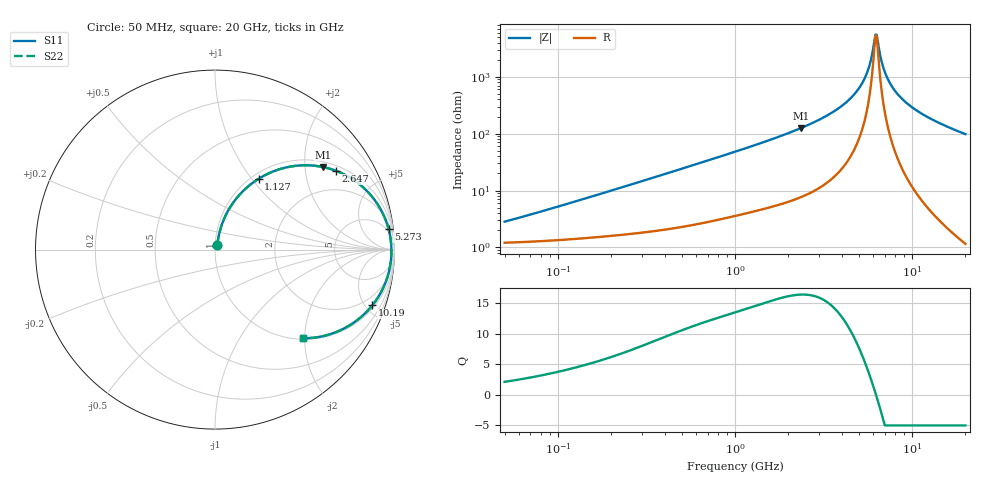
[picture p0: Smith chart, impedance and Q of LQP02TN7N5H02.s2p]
!Murata Part Number: LQP02TN7N5H02
!These Parameters are Measured in Series Mode Connection
!  o--[Z]--o
!Port1  Port2
!  o-------o
!Freq. Start=50[MHz] Stop=20[GHz], 401[Steps]
# Hz S RI R 50
!Freq.(Hz) S11(Real) S11(Imag) S21(Real) S21(Imag) S12(Real) S12(Imag) S22(Real) S22(Imag)
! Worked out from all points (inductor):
!   401 points, 50 MHz to 20 GHz, reference 50 ohm
!   read as one part in series: L = 8.03 nH near 76.05 MHz
!   highest Q = 16.4 at 2.349 GHz (marker M1), where L = 8.44 nH
!   self-resonance near 6.218 GHz
!   S11 on the Smith chart (normalised r, x): 50 MHz: 1.02, +0.05; 1.127 GHz: 1.08, +1.08; 2.647 GHz: 1.18, +2.93; 5.273 GHz: 4, +16; 10.19 GHz: 1.21, -5.57; 20 GHz: 1.02, -1.96
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5e7  0.0126 0.025  0.9874 -0.025  0.9874 -0.025  0.0126 0.025
1.364002e8  0.0186 0.0658  0.9814 -0.0658  0.9814 -0.0658  0.0186 0.0658
3.721004e8  0.049 0.1678  0.951 -0.1678  0.951 -0.1678  0.049 0.1678
1e9  0.2049 0.3682  0.7951 -0.3682  0.7951 -0.3682  0.2049 0.3682
1.127304e9  0.2435 0.3948  0.7565 -0.3948  0.7565 -0.3948  0.2435 0.3948
1.714689e9  0.4259 0.4635  0.5741 -0.4635  0.5741 -0.4635  0.4259 0.4635
2.348516e9  0.6029 0.4597  0.3971 -0.4597  0.3971 -0.4597  0.6029 0.4597
2.647493e9  0.6734 0.4393  0.3266 -0.4393  0.3266 -0.4393  0.6734 0.4393
2.728004e9  0.6909 0.4324  0.3091 -0.4324  0.3091 -0.4324  0.6909 0.4324
4.087748e9  0.8943 0.2697  0.1057 -0.2697  0.1057 -0.2697  0.8943 0.2697
4.748272e9  0.9437 0.1821  0.0563 -0.1821  0.0563 -0.1821  0.9437 0.1821
5.273168e9  0.967 0.1151  0.033 -0.1151  0.033 -0.1151  0.967 0.1151
5.683258e9  0.9774 0.0653  0.0226 -0.0653  0.0226 -0.0653  0.9774 0.0653
6.125241e9  0.9825 0.0146  0.0175 -0.0146  0.0175 -0.0146  0.9825 0.0146
6.217679e9  0.9829 0.00439  0.0171 -0.00439  0.0171 -0.00439  0.9829 0.00439
6.406762e9  0.983 -0.0161  0.017 0.0161  0.017 0.0161  0.983 -0.0161
6.905011e9  0.9794 -0.0671  0.0206 0.0671  0.0206 0.0671  0.9794 -0.0671
7.442007e9  0.9704 -0.1176  0.0296 0.1176  0.0296 0.1176  0.9704 -0.1176
8.516016e9  0.9408 -0.2052  0.0592 0.2052  0.0592 0.2052  0.9408 -0.2052
1.019291e10  0.8767 -0.3103  0.1233 0.3103  0.1233 0.3103  0.8767 -0.3103
1.375312e10  0.7205 -0.4386  0.2795 0.4386  0.2795 0.4386  0.7205 -0.4386
2e10  0.4902 -0.4941  0.5098 0.4941  0.5098 0.4941  0.4902 -0.4941
